(* Logix 5000 AddOnInstructionDefinition export RTA_435NBX_490NBX_PLC_to_Gateway; software revision 20.01 *)

TYPE RTA_STRING_4096 :   // string type; String Data Type with up to 4096 characters available
STRUCT
   LEN : DINT;
   DATA : SINT[4096];
END_STRUCT
END_TYPE

ADD_ON_INSTRUCTION RTA_435NBX_490NBX_PLC_to_Gateway   (* revision 1.0, vendor Real Time Automation, Inc. *)
// RTA's 435NBX / 490NBX PLC to Gateway handshaking
VAR_IN_OUT
   DataIn : RTA_STRING_4096; {required}
   DataOut : RTA_STRING_4096; {required}
END_VAR
VAR
   DataToGateway : RTA_STRING_4096; {access None}
   DataFromCustomer : RTA_STRING_4096; {access None}
   NULL_Tag : RTA_STRING_4096; {access None}
END_VAR

ROUTINE Logic   (* ladder *)
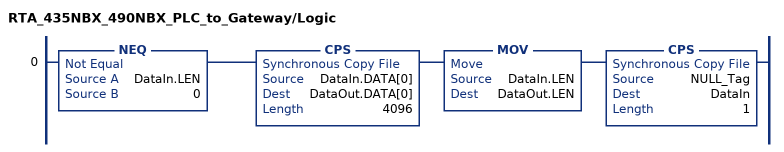
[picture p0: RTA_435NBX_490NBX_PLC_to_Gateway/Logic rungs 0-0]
   0: NEQ(DataIn.LEN,0)CPS(DataIn.DATA[0],DataOut.DATA[0],4096)MOV(DataIn.LEN,DataOut.LEN)CPS(NULL_Tag,DataIn,1);
END_ROUTINE
END_ADD_ON_INSTRUCTION
